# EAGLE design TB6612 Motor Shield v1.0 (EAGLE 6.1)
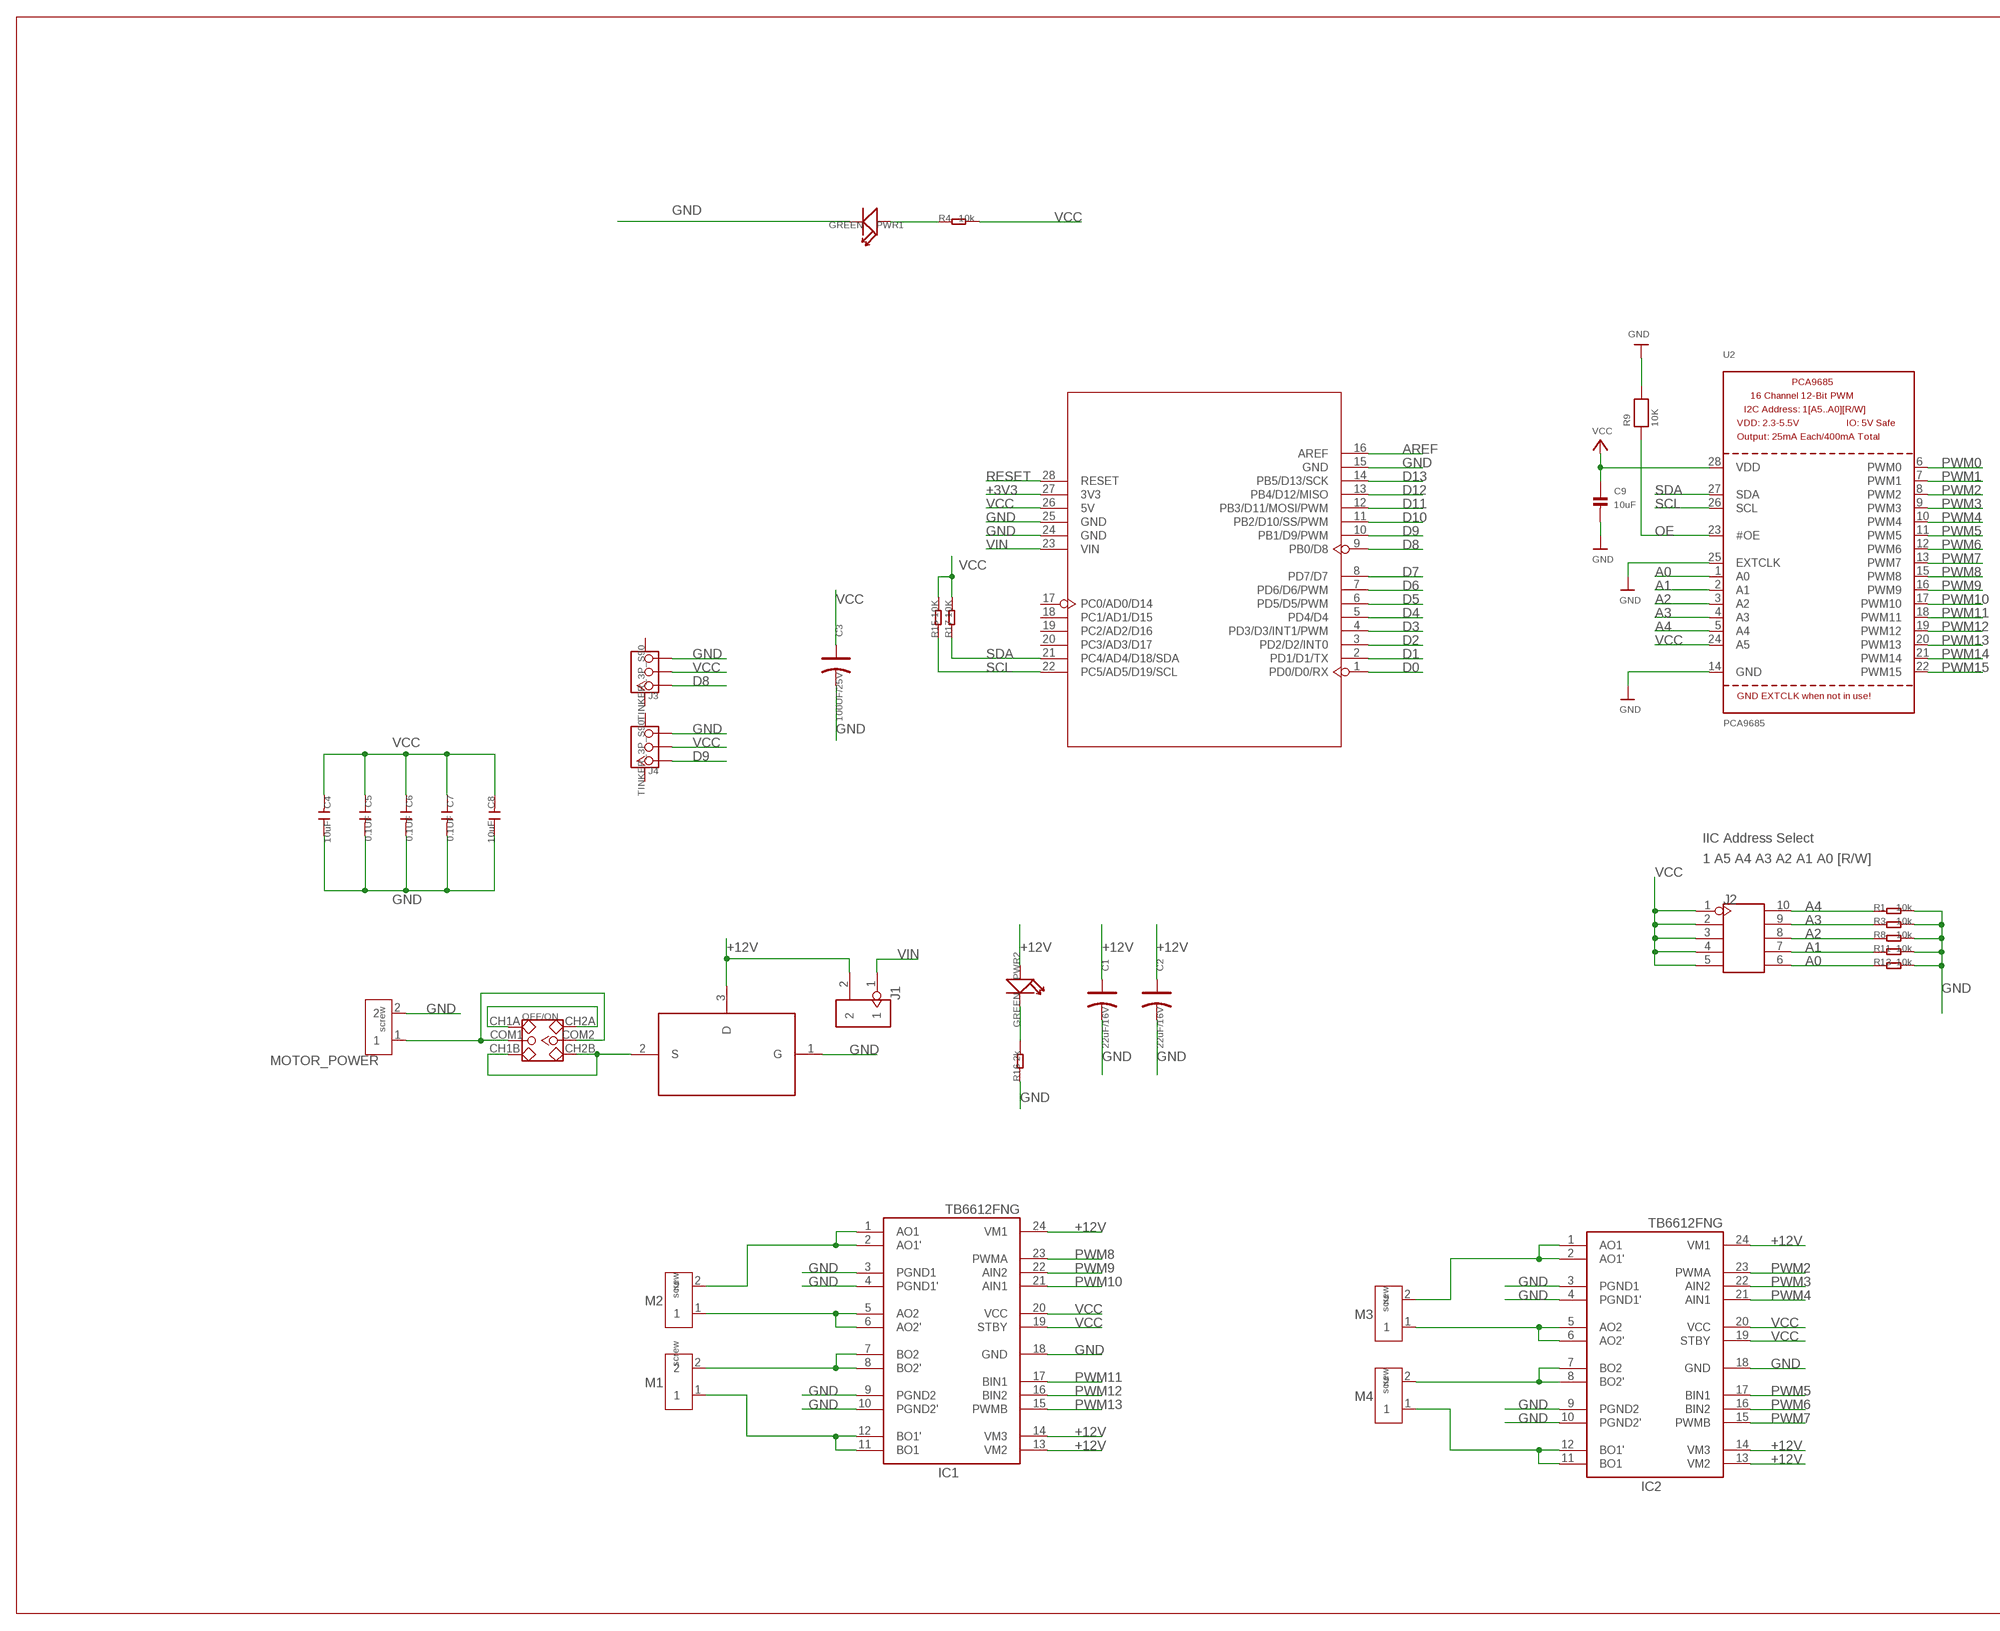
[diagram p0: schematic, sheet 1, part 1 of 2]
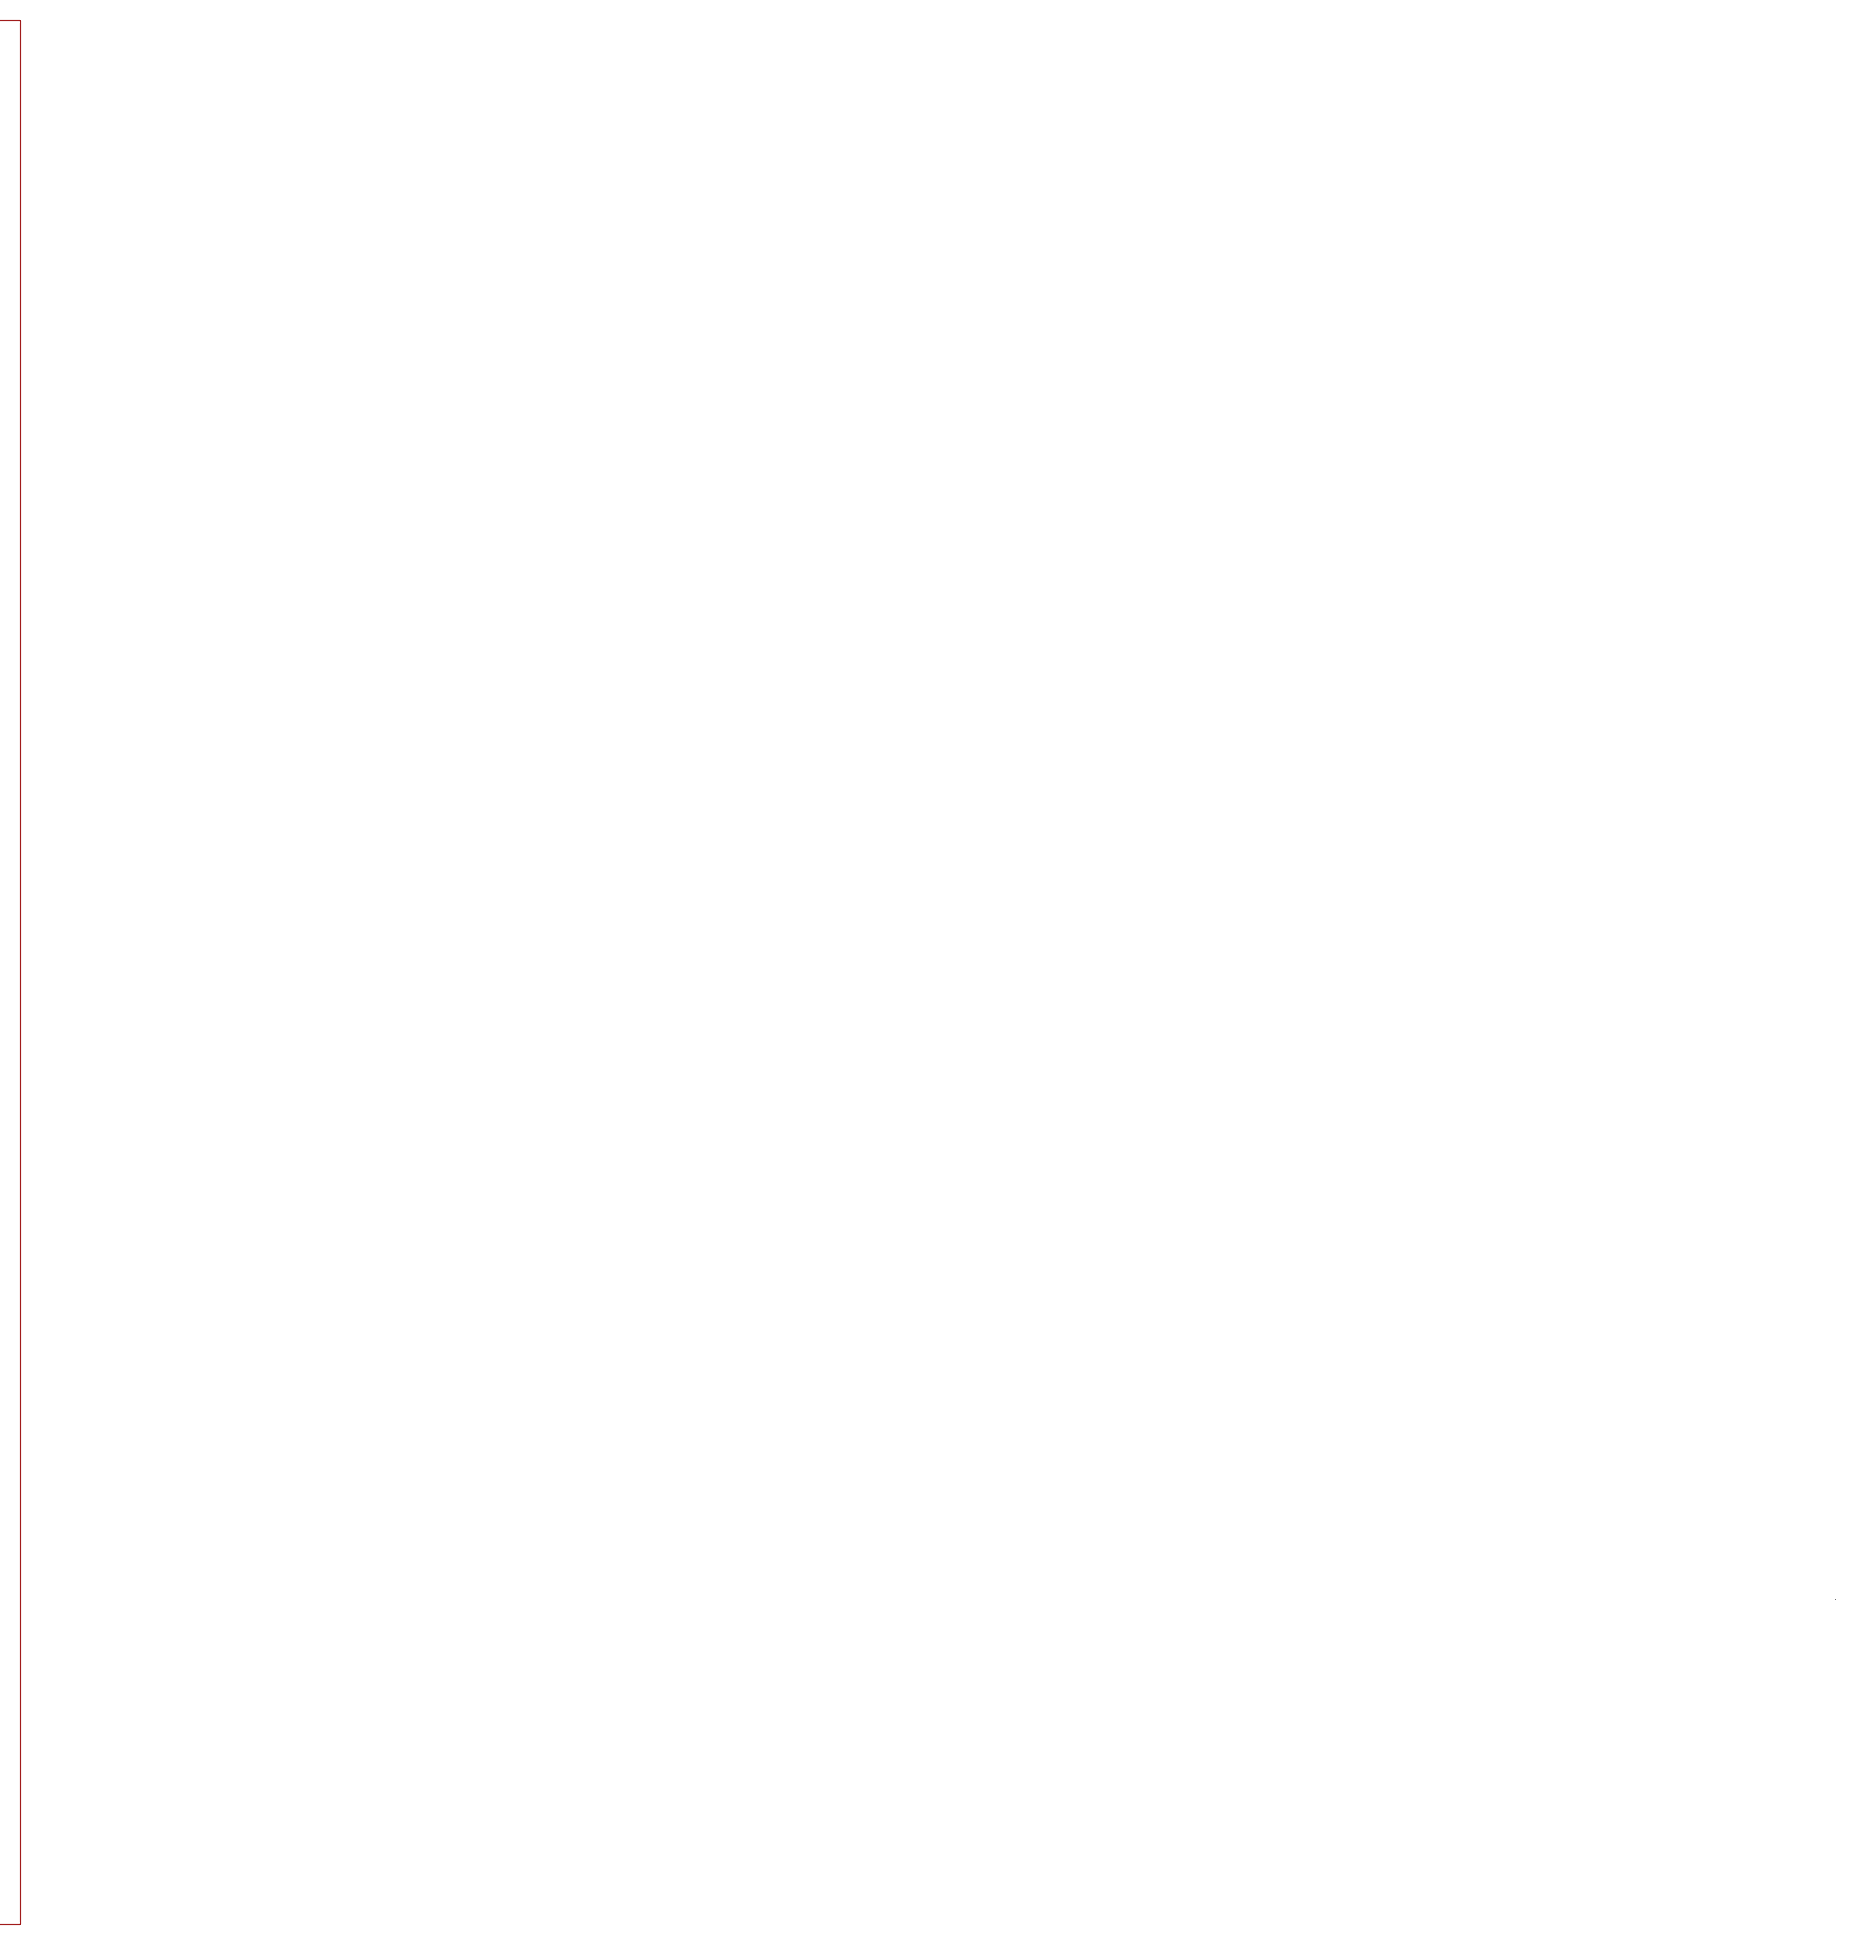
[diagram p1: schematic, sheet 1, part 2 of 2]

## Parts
C1  22uF/16V  CAP-ELECTRO-A  [ELECTRO-SMD-A-3.8MM]
C2  22uF/16V  CAP-ELECTRO-A  [ELECTRO-SMD-A-3.8MM]
C3  100UF/25V  CAP-ELECTRO-C  [ELECTRO-SMD-C-6MM]
C4  10uF  CAP-0805  [C0805]
C5  0.1UF  C-0603  [C0603]
C6  0.1UF  C-0603  [C0603]
C7  0.1UF  C-0603  [C0603]
C8  10uF  CAP-0805  [C0805]
C9  10uF  CAP_CERAMIC0805  [0805]
IC1  TB6612FNG  [SSOP24]
IC2  TB6612FNG  [SSOP24]
J1  HEADER-2P-65/35MIL  [2P-2.54-65/35MIL]
J2  HEADER-2X5P-2.54  [2X5P-2.54]
J3  TINKER_3P_S90  [TINKER_3P_S90]
J4  TINKER_3P_S90  [TINKER_3P_S90]
M1  screw  SCREW-TERMINAL-2P'5.0'  [2P-5.0]
M2  screw  SCREW-TERMINAL-2P'5.0'  [2P-5.0]
M3  screw  SCREW-TERMINAL-2P'5.0'  [2P-5.0]
M4  screw  SCREW-TERMINAL-2P'5.0'  [2P-5.0]
MOTOR_POWER  screw  SCREW-TERMINAL-2P'5.0'  [2P-5.0]
OFF/ON  SWITCH-2CH-6P  [6P-2CH-2.54-7.6X3.0]
PWR1  GREEN  LED'0603'  [LED-0603]
PWR2  GREEN  LED'0603'  [LED-0603]
R1  10k  R-0603  [R0603]
R3  10k  R-0603  [R0603]
R4  10k  R-0603  [R0603]
R8  10k  R-0603  [R0603]
R9  10K  RESISTOR0805  [0805]
R11  10k  R-0603  [R0603]
R13  10k  R-0603  [R0603]
R15  10K  R-0603  [R0603]
R16  2k  R-0603  [R0603]
R17  10K  R-0603  [R0603]
U1  AOD417  [AOD417]
U2  PCA9685  [TSSOP28]
U3  UNO-SHILED  [SHILED]

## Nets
+3V3: U3.27(3V3)
+12V: C1.+ C2.+ IC1.13(VM2) IC1.14(VM3) IC1.24(VM1) IC2.13(VM2) IC2.14(VM3) IC2.24(VM1) J1.2 PWR2.+ U1.3(D)
A0: J2.6 R13.1 U2.1(A0)
A1: J2.7 R11.1 U2.2(A1)
A2: J2.8 R8.1 U2.3(A2)
A3: J2.9 R3.1 U2.4(A3)
A4: J2.10 R1.1 U2.5(A4)
AREF: U3.16(AREF)
D0: U3.1(PD0/D0/RX)
D1: U3.2(PD1/D1/TX)
D2: U3.3(PD2/D2/INT0)
D3: U3.4(PD3/D3/INT1/PWM)
D4: U3.5(PD4/D4)
D5: U3.6(PD5/D5/PWM)
D6: U3.7(PD6/D6/PWM)
D7: U3.8(PD7/D7)
D8: J3.1 U3.9(PB0/D8)
D9: J4.1 U3.10(PB1/D9/PWM)
D10: U3.11(PB2/D10/SS/PWM)
D11: U3.12(PB3/D11/MOSI/PWM)
D12: U3.13(PB4/D12/MISO)
D13: U3.14(PB5/D13/SCK)
GND: C1.- C2.- C3.- C4.1 C5.2 C6.2 C7.2 C8.1 C9.2 IC1.3(PGND1) IC1.4(PGND1') IC1.9(PGND2) IC1.10(PGND2') IC1.18(GND) IC2.3(PGND1) IC2.4(PGND1') IC2.9(PGND2) IC2.10(PGND2') IC2.18(GND) J3.3 J4.3 MOTOR_POWER.2 PWR1.- R1.2 R3.2 R8.2 R9.2 R11.2 R13.2 R16.1 U1.1(G) U2.14(GND) U2.25(EXTCLK) U3.15(GND) U3.24(GND) U3.25(GND)
N$1: IC1.1(AO1) IC1.2(AO1') M2.2
N$2: IC1.5(AO2) IC1.6(AO2') M2.1
N$3: PWR1.+ R4.1
N$4: IC1.7(BO2) IC1.8(BO2') M1.2
N$5: IC1.11(BO1) IC1.12(BO1') M1.1
N$6: IC2.5(AO2) IC2.6(AO2') M3.1
N$7: IC2.1(AO1) IC2.2(AO1') M3.2
N$8: IC2.7(BO2) IC2.8(BO2') M4.2
N$9: OFF/ON.CH1B OFF/ON.CH2B U1.2(S)
N$10: IC2.11(BO1) IC2.12(BO1') M4.1
N$12: PWR2.- R16.2
N$13: MOTOR_POWER.1 OFF/ON.COM1 OFF/ON.COM2
N$15: OFF/ON.CH1A OFF/ON.CH2A
OE: R9.1 U2.23(#OE)
PWM0: U2.6(PWM0)
PWM1: U2.7(PWM1)
PWM2: IC2.23(PWMA) U2.8(PWM2)
PWM3: IC2.22(AIN2) U2.9(PWM3)
PWM4: IC2.21(AIN1) U2.10(PWM4)
PWM5: IC2.17(BIN1) U2.11(PWM5)
PWM6: IC2.16(BIN2) U2.12(PWM6)
PWM7: IC2.15(PWMB) U2.13(PWM7)
PWM8: IC1.23(PWMA) U2.15(PWM8)
PWM9: IC1.22(AIN2) U2.16(PWM9)
PWM10: IC1.21(AIN1) U2.17(PWM10)
PWM11: IC1.17(BIN1) U2.18(PWM11)
PWM12: IC1.16(BIN2) U2.19(PWM12)
PWM13: IC1.15(PWMB) U2.20(PWM13)
PWM14: U2.21(PWM14)
PWM15: U2.22(PWM15)
RESET: U3.28(RESET)
SCL: R15.1 U2.26(SCL) U3.22(PC5/AD5/D19/SCL)
SDA: R17.1 U2.27(SDA) U3.21(PC4/AD4/D18/SDA)
VCC: C3.+ C4.2 C5.1 C6.1 C7.1 C8.2 C9.1 IC1.19(STBY) IC1.20(VCC) IC2.19(STBY) IC2.20(VCC) J2.1 J2.2 J2.3 J2.4 J2.5 J3.2 J4.2 R4.2 R15.2 R17.2 U2.24(A5) U2.28(VDD) U3.26(5V)
VIN: J1.1 U3.23(VIN)
Unconnected: J3.SS1 J3.SS2 J4.SS1 J4.SS2 U3.17(PC0/AD0/D14) U3.18(PC1/AD1/D15) U3.19(PC2/AD2/D16) U3.20(PC3/AD3/D17)

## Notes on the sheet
- IIC Address Select
- 1 A5 A4 A3 A2 A1 A0 [R/W]

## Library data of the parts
C1-C3 = Discrete:CAP*: Electrolytic Capacitors,Tantalum Capacitors and Super Capacitors
C4 C8 = Discrete-new:CAP: Ceramic Capacitors
C5-C7 = Discrete:C*: Ceramic Capacitors
C9 = microbuilder:CAP_CERAMIC: Ceramic Capacitors
IC1 IC2 = adafruit:TB6612FNG: TB6612FNG MOS dual H-bridge motor driver, 1.2A current 3.2A peak 3 or 5v logic and 3-15v motor
J1 = Connector:HEADER-2P
J2 = Connector:HEADER-2X5P
J3 J4 = Connector:TINKER_3P_S90
M1-M4 MOTOR_POWER = Connector:SCREW-TERMINAL-2P
OFF/ON = Discrete:SWITCH-2CH-6P
PWR1 PWR2 = Discrete:LED*
R1 R3 R4 R8 R11 R13 R15-R17 = Discrete:R*
R9 = microbuilder:RESISTOR: Resistors
U1 = aod417:AOD417
U2 = microbuilder:PCA9685: PCA9685 - 16 Channel 12-Bit I2C PWM Controller 5.0V tolerant 16 channel, 12-bit I2C PWM controller with 25mA per output (max. 400mA total) Digikey: 568-5931-1-ND
U3 = ljb:UNO-SHILED

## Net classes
2 gnd: width 0.305 mm, drill 0.559 mm, clearance 0.254 mm

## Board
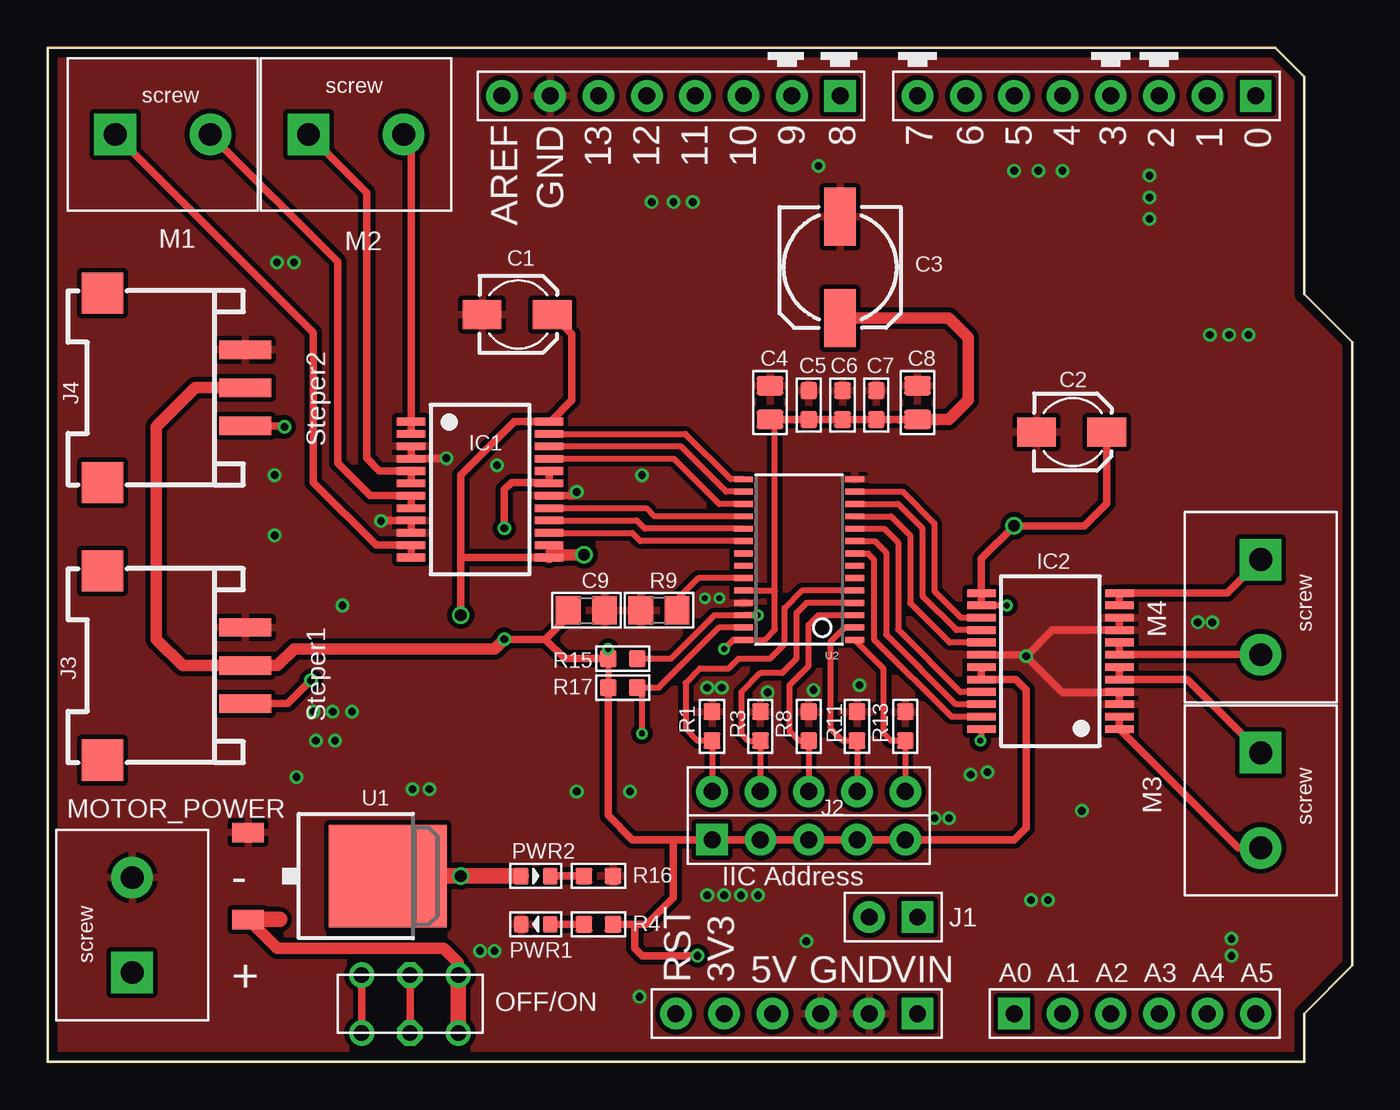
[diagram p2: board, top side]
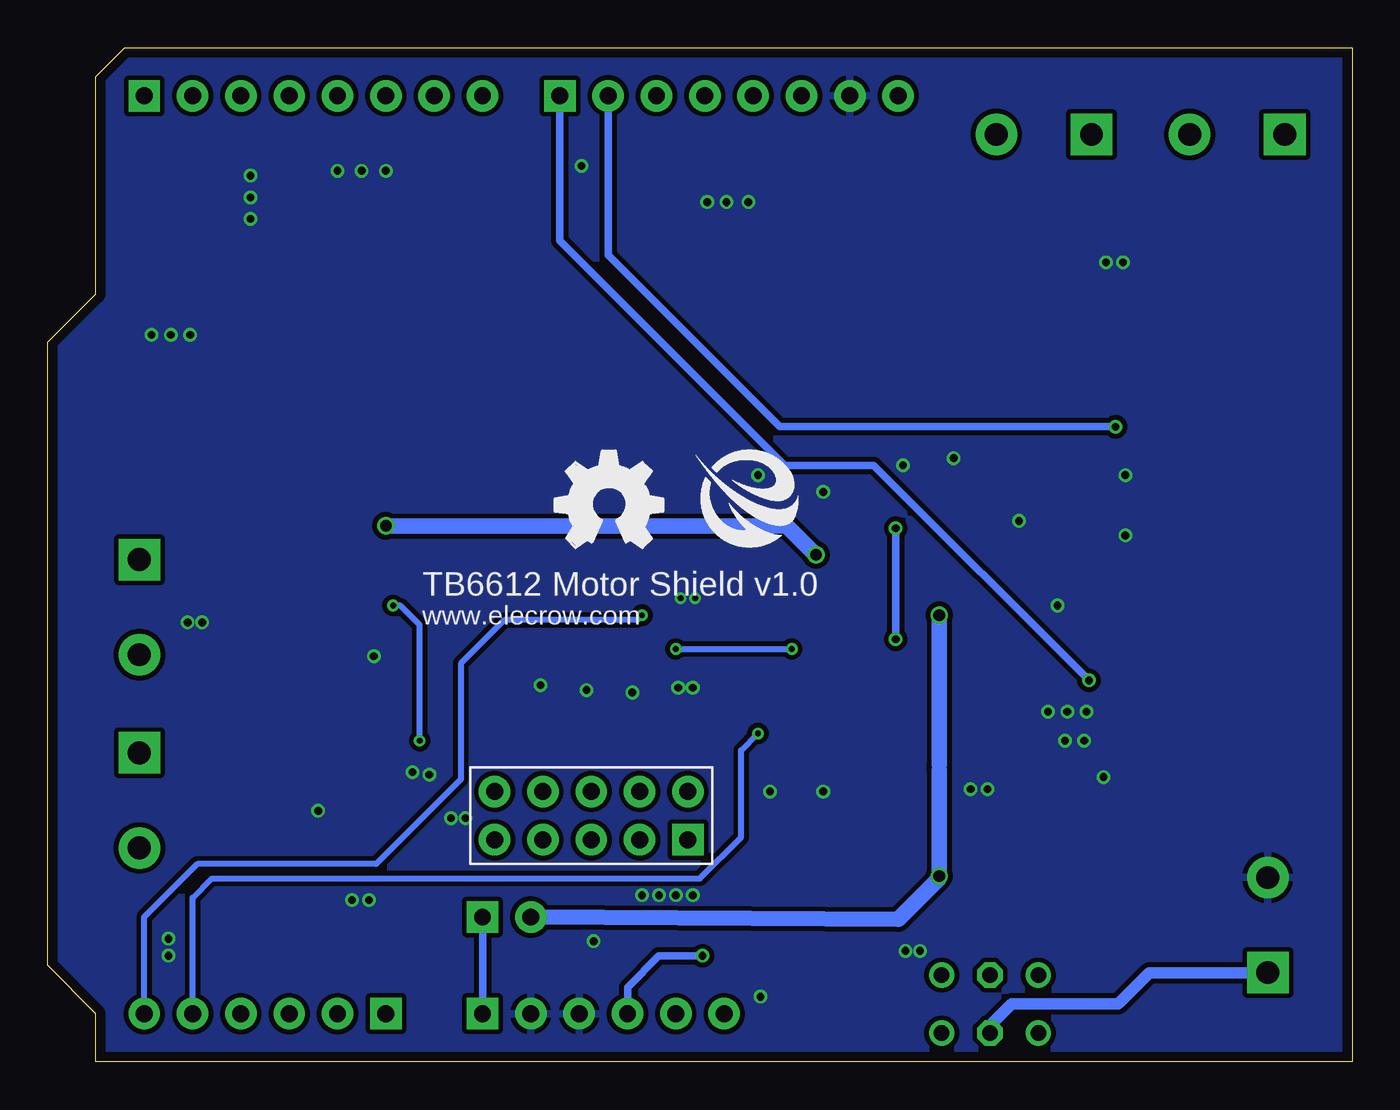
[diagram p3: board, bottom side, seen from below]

Size 68.58 x 53.34 mm. Coordinates in mm from the lower left corner, seen from the top.
Outline: 0,0 66.04,0 66.04,2.54 68.58,5.08 68.58,37.85 66.04,40.39 66.04,51.82 64.52,53.34 0,53.34 0,0
Copper layers (1*16): Top 0.035mm / dielectric 1.5mm / Bottom 0.035mm
Design rules: minimum track width 10mil, minimum drill 12mil, track to track 8mil, track to pad 8mil, pad to pad 8mil, via to via 8mil, smd to smd 0mil, copper to edge 20mil, drill to drill 10mil, minimum pad ring 10mil, minimum via ring 6mil, stop-mask expansion 2mil, vias tented up to drill 100mil, thermal gap 10mil

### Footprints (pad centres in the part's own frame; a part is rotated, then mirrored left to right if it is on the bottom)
ELECTRO-SMD-A-3.8MM = smd 2.032 x 1.524: + 1.778,0; - -1.905,0
ELECTRO-SMD-C-6MM = smd 3.048 x 1.651: + 2.667,0; - -2.667,0
C0805 = smd 1.397 x 1.016: 1 0,0.889; 2 0,-0.889
C0603 = smd 0.889 x 0.889: 1 -0.762,0; 2 0.762,0
0805 = smd 1.3 x 1.5: 1 -0.95,0; 2 0.95,0
SSOP24 = smd 0.4 x 1.5: 1 -3.575,-3.625; 2 -2.925,-3.625; 3 -2.275,-3.625; 4 -1.625,-3.625; 5 -0.975,-3.625; 6 -0.325,-3.625; 7 0.325,-3.625; 8 0.975,-3.625; 9 1.625,-3.625; 10 2.275,-3.625; 11 2.925,-3.625; 12 3.575,-3.625; 13 3.575,3.625; 14 2.925,3.625; 15 2.275,3.625; 16 1.625,3.625; 17 0.975,3.625; 18 0.325,3.625; 19 -0.325,3.625; 20 -0.975,3.625; 21 -1.625,3.625; 22 -2.275,3.625; 23 -2.925,3.625; 24 -3.575,3.625
2P-2.54-65/35MIL = drill 0.889 pad 1.651 square: 1 0,1.27 | drill 0.889 pad 1.651: 2 0,-1.27
2X5P-2.54 = drill 0.889 pad 1.651 square: 1 -1.27,5.08 | drill 0.889 pad 1.651: 2 -1.27,2.54; 3 -1.27,0; 4 -1.27,-2.54; 5 -1.27,-5.08; 6 1.27,-5.08; 7 1.27,-2.54; 8 1.27,0; 9 1.27,2.54; 10 1.27,5.08
TINKER_3P_S90 = smd 0.965 x 2.74: 1 -1.984,-4.545; 2 0.016,-4.545; 3 2.016,-4.545 | smd 2.159 x 2.184: SS1 -4.958,2.955; SS2 4.99,2.955
2P-5.0 = drill 1.2 pad 2.184 square: 1 0,0 | drill 1.2 pad 2.184: 2 5,0
6P-2CH-2.54-7.6X3.0 = drill 0.813 pad 1.27: CH1A -1.524,2.54; CH1B -1.524,-2.54; CH2A 1.524,2.54; CH2B 1.524,-2.54 | drill 0.813 pad 1.27 octagon: COM1 -1.524,0; COM2 1.524,0
LED-0603 = smd 0.762 x 0.889: + -0.762,0; - 0.762,0
R0603 = smd 0.889 x 0.889: 1 -0.762,0; 2 0.762,0
AOD417 = smd 1.016 x 1.651: 1 -2.286,-6.096; 2 2.286,-6.096 | smd 5.4 x 6.2: 3 0,1.23
TSSOP28 = smd 0.305 x 0.991: 1 -4.225,-2.918; 2 -3.575,-2.918; 3 -2.925,-2.918; 4 -2.275,-2.918; 5 -1.625,-2.918; 6 -0.975,-2.918; 7 -0.325,-2.918; 8 0.325,-2.918; 9 0.975,-2.918; 10 1.625,-2.918; 11 2.275,-2.918; 12 2.925,-2.918; 13 3.575,-2.918; 14 4.225,-2.918; 15 4.225,2.918; 16 3.575,2.918; 17 2.925,2.918; 18 2.275,2.918; 19 1.625,2.918; 20 0.975,2.918; 21 0.325,2.918; 22 -0.325,2.918; 23 -0.975,2.918; 24 -1.625,2.918; 25 -2.275,2.918; 26 -2.925,2.918; 27 -3.575,2.918; 28 -4.225,2.918
SHILED = drill 0.889 pad 1.651 square: 1 63.5,50.8; 9 41.656,50.8; 17 50.8,2.54; 23 45.72,2.54 | drill 0.889 pad 1.651: 2 60.96,50.8; 3 58.42,50.8; 4 55.88,50.8; 5 53.34,50.8; 6 50.8,50.8; 7 48.26,50.8; 8 45.72,50.8; 10 39.116,50.8; 11 36.576,50.8; 12 34.036,50.8; 13 31.496,50.8; 14 28.956,50.8; 15 26.416,50.8; 16 23.876,50.8; 18 53.34,2.54; 19 55.88,2.54; 20 58.42,2.54; 21 60.96,2.54; 22 63.5,2.54; 24 43.18,2.54; 25 40.64,2.54; 26 38.1,2.54; 27 35.56,2.54; 28 33.02,2.54

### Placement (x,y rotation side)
C1  24.75,39.31 0 top
C2  53.89,33.12 0 top
C3  41.66,41.78 270 top
C4  37.97,34.67 0 top
C5  40.01,34.54 90 top
C6  41.78,34.54 90 top
C7  43.56,34.54 90 top
C8  45.72,34.67 0 top
C9  28.32,23.75 0 top
IC1  22.73,30.1 270 top
IC2  52.7,21.08 90 top
J1  44.45,7.62 270 top
J2  40.01,12.95 90 top
J3  5.84,20.83 90 top
J4  5.84,35.43 90 top
LOGO2  LOGO-OSHW-FILLX0200-NT  [OSHW_FILLX200_NOTEXT]  41.91,27.05 0 bottom
M1  3.56,48.77 0 top
M2  13.72,48.77 0 top
M3  63.75,16.26 270 top
M4  63.75,26.42 270 top
MOTOR_POWER  4.45,4.7 90 top
OFF/ON  19.05,3.05 90 top
PWR1  25.65,7.24 180 top
PWR2  25.65,9.78 0 top
R1  34.92,17.65 90 top
R3  37.47,17.65 90 top
R4  28.96,7.24 0 top
R8  40.01,17.65 90 top
R9  32.13,23.75 180 top
R11  42.55,17.65 90 top
R13  45.09,17.65 90 top
R15  30.23,21.21 180 top
R16  28.96,9.78 180 top
R17  30.23,19.68 180 top
U1  16.64,9.78 270 top
U2  39.5,26.42 90 top
U3  0,0 0 top
U$1  [ELECROW-NEW]  34.54,27.05 0 bottom

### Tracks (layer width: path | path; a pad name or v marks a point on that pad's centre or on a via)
+12V  (via drill 0.3, 0.61)
  Top 0.305: IC2.24 49.08,16.95 v49.02,16.89 | v50.42,24 IC2.14
  Top 0.406: IC1.14 IC1.13 21.74,26.52 21.72,26.54 | v50.8,28.19 49.08,26.47 IC2.13 IC2.14 49.02,24.01 | 49.15,26.54 v50.8,28.19 | 21.72,26.54 v21.72,23.5 | 21.72,26.54 21.72,30.86 24.53,33.67 IC1.24 26.43,33.67 27.56,34.8 27.56,38.27 C1.+ | v50.8,28.19 54.48,28.19 55.66,29.38 C2.+
  Top 0.61: v28.19,26.67 26.5,26.67 IC1.13
  Top 0.813: U1.3 v21.72,9.78 PWR2.+
  Bottom 0.305: v49.02,16.89 49.02,22.99 50.04,24 v50.42,24
  Bottom 0.406: v21.72,9.78 21.72,9.65
  Bottom 0.61: 21.72,15.37 21.72,15.62
  Bottom 0.813: v21.72,23.5 21.72,15.62 | 21.72,15.37 v21.72,9.78 | J1.2 23.88,7.49 21.72,9.65 | v50.8,28.19 29.72,28.19 v28.19,26.67
A0
  Top 0.305: J2.6 R13.1 44.32,16.89 43.94,17.27 43.94,20.66 U2.1
A1
  Top 0.305: U2.2 41.89,22.84 41.15,22.1 41.15,17.53 41.78,16.89 R11.1 J2.7
A2
  Top 0.305: U2.3 40.51,23.49 40.01,22.99 40.01,20.83 38.99,19.81 38.99,17.4 39.5,16.89 R8.1 J2.8
A3
  Top 0.305: J2.9 R3.1 36.83,16.89 36.45,17.27 36.45,19.43 37.47,20.45 38.61,20.45 39.37,21.21 39.37,23.62 39.89,24.14 U2.4
A4
  Top 0.305: J2.10 R1.1 34.16,16.89 33.53,17.53 33.53,19.94 34.29,20.7 35.81,20.7 36.32,21.21 37.97,21.21 38.73,21.97 38.73,23.88 39.65,24.79 U2.5
D8  (via drill 0.41)
  Top 0.406: J3.1 12.62,18.84 v13.84,20.07
  Bottom 0.406: U3.9 41.66,43.18 29.84,31.37 25.15,31.37 v13.84,20.07
D9  (via drill 0.41)
  Top 0.406: J4.1 12.4,33.45 v12.45,33.4
  Bottom 0.406: U3.10 39.12,42.42 30.1,33.4 v12.45,33.4
GND  (via drill 0.3, 0.41)
  Top 0.406: IC1.3 IC1.4 20.93,31.72 v20.95,31.75 | IC1.10 IC1.9 17.43,28.47 v17.53,28.45 | IC2.18 51.44,21.41 v51.44,21.34 | IC2.10 IC2.9 52.81,22.71 v51.44,21.34 | IC2.3 56.39,18.81 56.39,18.8 56.33,18.8 IC2.4 56.29,19.46 56.26,19.43 53.34,19.43 v51.44,21.34 | IC1.18 27.61,29.77 v27.81,29.97
  other vias: 11.94,30.86 34.67,8.76 13.97,18.41 35.56,8.76 40.51,47.12 13.08,14.99 36.45,8.76 50.8,46.86 16,18.41 30.61,14.22 32.89,45.21 12.95,42.04 33.91,45.21 60.45,23.11 61.09,38.23 52.07,46.86 31.75,45.21 63.12,38.23 51.69,8.51 53.34,46.86 20.07,14.35 19.18,14.35 22.73,5.84 15.11,16.89 57.91,45.47 57.91,44.32 37.34,8.76 57.91,46.61 52.58,8.51 23.5,5.84 14.1,16.89 14.99,18.41 12.06,42.04 62.1,38.23 11.94,27.69 15.49,24 61.21,23.11 27.81,14.22 39.88,6.35 31.11,3.43 54.36,13.21 31.24,30.86 23.62,31.37 34.67,19.68 37.85,19.43 40.26,19.56 42.67,19.81 35.43,19.68 34.54,24.38 35.31,24.38 48.51,15.11 49.4,15.24 46.61,12.83 47.37,12.83 62.23,6.48 62.23,5.59
  pour Bottom (isolate 0.254): -1.27,-1.27 71.12,-1.27 71.12,54.61 -1.27,54.61
  pour Top (isolate 0.254): -1.27,-1.27 71.12,-1.27 71.12,54.61 -1.27,54.61
N$1
  Top 0.406: IC1.2 IC1.1 19.11,48.38 M2.2
N$2
  Top 0.406: IC1.6 IC1.5 17.44,31.07 16.76,31.75 16.76,45.72 M2.1
N$3
  Top 0.406: PWR1.+ R4.1
N$4
  Top 0.406: IC1.8 IC1.7 16.96,29.77 15.24,31.5 15.24,42.08 M1.2
N$5
  Top 0.406: IC1.12 IC1.11 17.28,27.17 13.97,30.48 13.97,38.35 M1.1
N$6
  Top 0.406: IC2.6 IC2.5 59.9,20.11 M3.1
N$7
  Top 0.406: IC2.2 IC2.1 62.58,11.26 M3.2
N$8
  Top 0.406: IC2.8 IC2.7 M4.2
N$9
  Top 0.61: OFF/ON.CH2B 21.59,5.21 20.83,5.97 12.06,5.97 U1.2
  Top 0.813: OFF/ON.CH1B OFF/ON.CH2B | 12.19,7.49 U1.2
N$10
  Top 0.406: M4.1 61.99,24.66 IC2.12 IC2.11
N$12
  Top 0.406: PWR2.- R16.2
N$13
  Top 0.406: OFF/ON.COM1 OFF/ON.COM2
  Bottom 0.61: MOTOR_POWER.1 10.67,4.7 12.32,3.05 17.91,3.05 19.05,1.91 OFF/ON.COM1
N$15
  Top 0.406: OFF/ON.CH1A OFF/ON.CH2A
OE
  Top 0.305: U2.23 34.2,25.44 33.08,24.32 R9.1
PWM2
  Top 0.305: U2.8 43.11,26.74 43.43,26.42 43.43,22.23 47.5,18.16 IC2.23
PWM3
  Top 0.305: U2.9 43.48,27.39 44.07,26.8 44.07,22.48 47.74,18.81 IC2.22
PWM4
  Top 0.305: U2.10 43.97,28.04 44.7,27.3 44.7,22.73 47.98,19.46 IC2.21
PWM5
  Top 0.305: U2.11 44.33,28.69 45.34,27.69 45.34,24.13 47.41,22.06 IC2.17
PWM6
  Top 0.305: U2.12 44.7,29.34 45.97,28.07 45.97,24.51 47.78,22.71 IC2.16
PWM7
  Top 0.305: U2.13 44.94,29.99 46.61,28.32 46.61,24.77 48.02,23.36 IC2.15
PWM8
  Top 0.305: IC1.23 33.52,33.02 35.91,30.64 U2.15
PWM9
  Top 0.305: IC1.22 33.28,32.37 35.67,29.99 U2.16
PWM10
  Top 0.305: IC1.21 32.92,31.72 35.31,29.34 U2.17
PWM11
  Top 0.305: U2.18 31.89,28.69 31.45,29.12 IC1.17
PWM12
  Top 0.305: U2.19 31.39,28.04 30.96,28.47 IC1.16
PWM13
  Top 0.305: U2.20 31.16,27.39 30.72,27.82 IC1.15
SCL  (via drill 0.3)
  Top 0.305: R15.1 32.77,21.21 35.05,23.49 U2.26 v37.34,23.5
  Bottom 0.305: U3.22 63.5,7.62 60.71,10.41 51.31,10.41 46.86,14.86 46.86,20.95 44.58,23.24 37.59,23.24 v37.34,23.5
SDA  (via drill 0.3)
  Top 0.305: U2.27 35.29,22.84 32.13,19.68 R17.1 31.24,19.43 v31.24,17.27
  Bottom 0.305: U3.21 60.96,8.64 59.94,9.65 34.29,9.65 32.13,11.81 32.13,16.38 v31.24,17.27
VCC  (via drill 0.3, 0.41)
  Top 0.305: R17.2 R15.2 v29.46,21.72 | 38.23,24.77 38.23,22.73 37.69,22.19 U2.28 36.03,22.19 v35.56,21.72 | 38.23,24.77 38.23,33.4 38.61,33.78 | U2.24 38.2,24.79 38.23,24.77
  Top 0.406: IC2.19 IC2.20 50.89,20.11 51.44,19.56 51.44,12.32 50.8,11.68 J2.5 J2.4 J2.3 J2.2 J2.1 33.02,11.68 | IC1.20 IC1.19 26.3,30.48 24.38,30.48 24,30.1 v24,28.07 | C4.2 38.61,33.78 C5.1 C6.1 C7.1 C8.2 45.85,33.66 | v24,22.23 26.16,22.23 | 26.16,22.23 27.37,23.43 C9.1 | R15.2 27.18,21.21 26.16,22.23 | 33.02,11.68 30.73,11.68 29.46,12.95 R17.2 | R4.2 30.99,7.24 | 30.99,7.24 31.5,7.24 32.89,8.64 32.89,11.56 33.02,11.68 | v34.16,5.59 31.24,5.59 30.86,5.97 30.86,7.11 30.99,7.24
  Top 0.61: J4.2 7.76,35.45 5.71,33.4 5.71,22.23 7.1,20.84 J3.2 12.08,20.84 12.95,21.72 23.5,21.72 v24,22.23 | C3.+ 47.37,39.12 48.39,38.1 48.39,34.8 47.37,33.78 C8.2
  Bottom 0.305: v35.56,21.72 v29.46,21.72
  Bottom 0.406: v24,28.07 v24,22.23 | U3.26 38.1,3.94 36.45,5.59 v34.16,5.59
VIN
  Bottom 0.406: J1.1 U3.23

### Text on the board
tPlace: 13 | 12 | 11 | 10 | 9 | 8 | 7 | 6 | 5 | 4 | 3 | 2 | 1 | 0
bPlace: TB6612 Motor Shield v1.0 | www.elecrow.com
tNames: AREF | GND | Steper2 | Steper1 | - | IIC Address | + | RST | 3V3 | 5V | GND | VIN | A0 | A1 | A2 | A3 | A4 | A5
